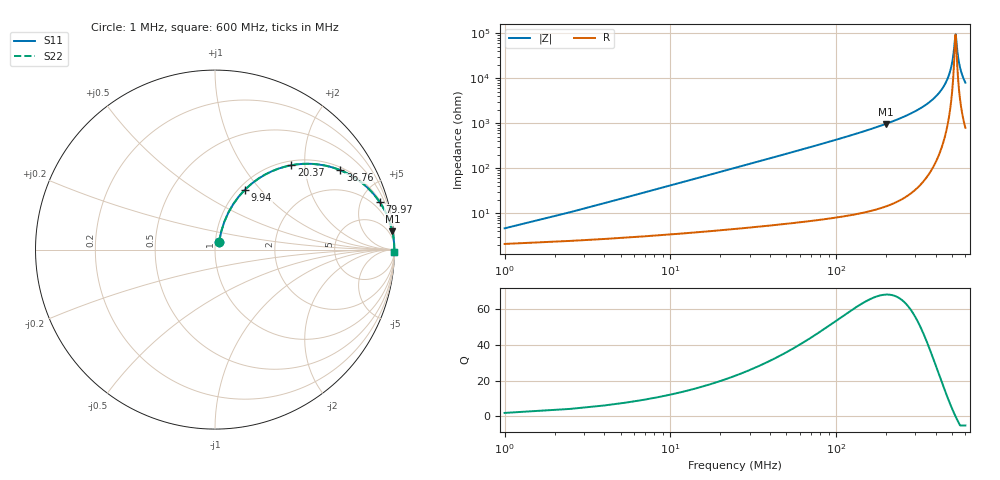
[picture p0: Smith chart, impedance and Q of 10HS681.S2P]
! Coilcraft 1008HS-681 Chip Inductor
! 02 July 2002
# MHZ S MA R 50
!Freq  MagS11  AngS11  MagS21  AngS21  MagS12  AngS12  MagS22  AngS22
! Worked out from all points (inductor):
!   404 points, 1 MHz to 600 MHz, reference 50 ohm
!   read as one part in series: L = 665 nH near 3.98 MHz
!   highest Q = 67.9 at 199.2 MHz (marker M1), where L = 778 nH
!   self-resonance near 522.5 MHz
!   S11 on the Smith chart (normalised r, x): 1 MHz: 1.04, +0.08; 9.94 MHz: 1.07, +0.83; 20.37 MHz: 1.09, +1.70; 36.76 MHz: 1.10, +3.09; 79.97 MHz: 1.14, +6.84; 600 MHz: open
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1  0.0458 60.9  0.9785 -2.3  0.9785 -2.3  0.0458 60.9
5.47  0.2186 70.2  0.9485 -12.5  0.9485 -12.5  0.2186 70.2
9.94  0.374 63.4  0.8972 -21.9  0.8972 -21.9  0.374 63.4
20.37  0.6337 47.9  0.7425 -39.3  0.7425 -39.3  0.6337 47.9
36.76  0.8267 32.3  0.5353 -55.7  0.5353 -55.7  0.8267 32.3
54.64  0.9089 23.2  0.3936 -65.3  0.3936 -65.3  0.9089 23.2
79.97  0.9544 16.2  0.2789 -72.6  0.2789 -72.6  0.9544 16.2
102.32  0.9718 12.6  0.2186 -76.3  0.2186 -76.3  0.9718 12.6
199.17  0.9933 5.9  0.1021 -83.3  0.1021 -83.3  0.9933 5.9
202.15  0.9935 5.7  0.1001 -83.4  0.1001 -83.4  0.9935 5.7
301.98  0.9976 3.0  0.05276 -85.9  0.05276 -85.9  0.9976 3.0
401.81  0.9988 1.4  0.02446 -86.5  0.02446 -86.5  0.9988 1.4
464.39  0.999 0.6  0.01102 -84.4  0.01102 -84.4  0.999 0.6
485.25  0.999 0.4  0.007013 -81.5  0.007013 -81.5  0.999 0.4
501.64  0.999 0.2  0.004035 -75.1  0.004035 -75.1  0.999 0.2
510.58  0.999 0.1  0.002514 -65.5  0.002514 -65.5  0.999 0.1
519.52  0.9989 0.0  0.001269 -33.7  0.001269 -33.7  0.9989 0.0
523.99  0.9989 -0.0  0.001068 4.1  0.001068 4.1  0.9989 -0.0
540.38  0.9989 -0.2  0.003092 69.0  0.003092 69.0  0.9989 -0.2
552.3  0.9989 -0.3  0.005012 76.7  0.005012 76.7  0.9989 -0.3
573.16  0.9988 -0.5  0.008359 81.4  0.008359 81.4  0.9988 -0.5
600  0.9987 -0.7  0.01254 83.5  0.01254 83.5  0.9987 -0.7
